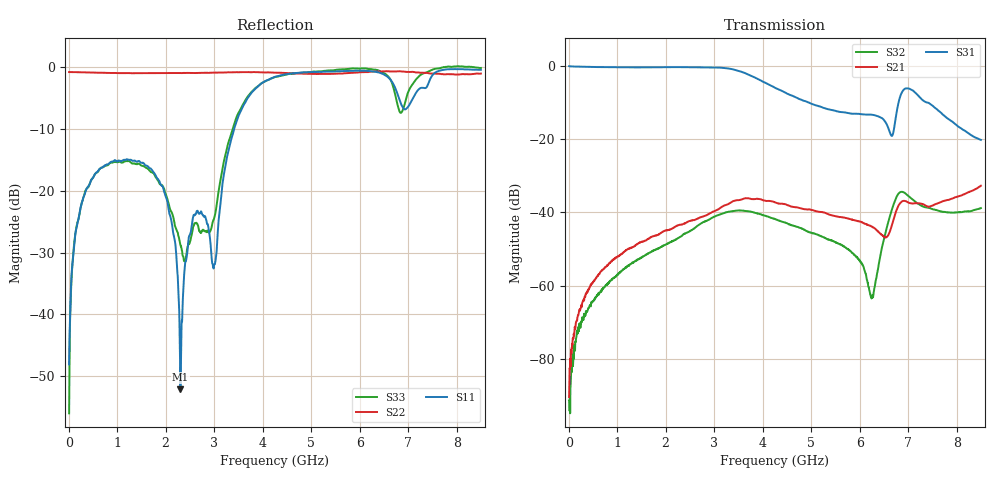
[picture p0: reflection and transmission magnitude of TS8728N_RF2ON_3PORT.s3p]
!Created with skrf (http://scikit-rf.org).
# GHz S RI R 50.0
!freq ReS11 ImS11 ReS12 ImS12 ReS13 ImS13
! ReS21 ImS21 ReS22 ImS22 ReS23 ImS23
! ReS31 ImS31 ReS32 ImS32 ReS33 ImS33
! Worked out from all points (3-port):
!   1601 points, 10 MHz to 8.5 GHz, reference 50 ohm
!   strongest paths, dB at 10 MHz, 2.132 GHz, 4.255 GHz, 6.378 GHz, 8.5 GHz:
!     S31: -0.1, -0.3, -6.0, -13.7, -20.2
!     S21: -90.4, -44.4, -37.2, -45.2, -32.7
!     S32: -91.3, -47.9, -41.8, -55.6, -38.8
!   lowest |S11| = -52.1 dB at 2.302 GHz (marker M1), VSWR 1.00, Z = 49.8 + j0.179 ohm
!   |S11| at or under -10 dB: start of sweep to 3.412 GHz
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0.01  0.0039 0.000434  1.92e-05 3.12e-05  0.9932 -0.0102
      8.58e-06 2.88e-05  -0.9168 0.00505  1.74e-05 -8.1e-06
      0.9933 -0.0103  2.66e-05 5.28e-06  0.00138 0.000765
0.2965375  -0.00946 -0.0858  -3.48e-05 0.00062  0.9652 -0.1427
           -3.81e-05 0.000619  -0.9083 0.0859  -9.57e-05 -0.000336
           0.9654 -0.1428  -0.000132 -0.000325  -0.0071 -0.0859
1.182681  -0.0979 -0.1496  -0.00036 0.00303  0.8142 -0.5018
          -0.000384 0.00305  -0.8193 0.3704  -0.00173 -0.00039
          0.8141 -0.5019  -0.00171 -0.000364  -0.0726 -0.1582
1.983925  -0.0796 -0.0512  -0.00018 0.00563  0.5688 -0.7754
          -0.000171 0.00564  -0.7233 0.5369  -0.00335 0.0014
          0.5687 -0.7756  -0.00331 0.00138  -0.05 -0.0852
2.3023  -0.0017 0.0018  0.000128 0.0068  0.427 -0.8645
        8.72e-05 0.00681  -0.6687 0.6038  -0.00394 0.00246
        0.427 -0.8645  -0.00391 0.00251  0.0112 -0.0349
4.255  -0.6353 0.549  0.011 0.00823  -0.3936 -0.3151
       0.011 0.00823  -0.2203 0.8807  0.00654 0.00478
       -0.3937 -0.3139  0.00655 0.00478  -0.332 0.7684
6.25015  -0.6251 0.6903  0.00555 0.00322  -0.1763 -0.1248
         0.00553 0.00324  0.3738 0.8448  0.000163 0.00068
         -0.1763 -0.1245  0.000142 0.00069  -0.4261 0.8666
6.823225  0.3076 0.4516  0.00187 0.013  -0.0569 -0.3543
          0.00187 0.013  0.4888 0.7917  -0.00216 0.0185
          -0.0568 -0.3542  -0.00221 0.0185  0.4315 -0.0814
7.406912  0.2351 -0.6844  0.00735 0.00949  -0.3122 0.0455
          0.00737 0.00941  0.5498 0.7121  0.00948 0.00665
          -0.3125 0.0461  0.00948 0.00671  -0.7156 -0.5805
8.5  -0.0119 -0.9563  0.0163 0.0163  -0.0898 0.0376
     0.0164 0.0163  0.7928 0.4073  0.0106 0.0043
     -0.0901 0.0381  0.0106 0.00433  -0.6564 -0.7413
